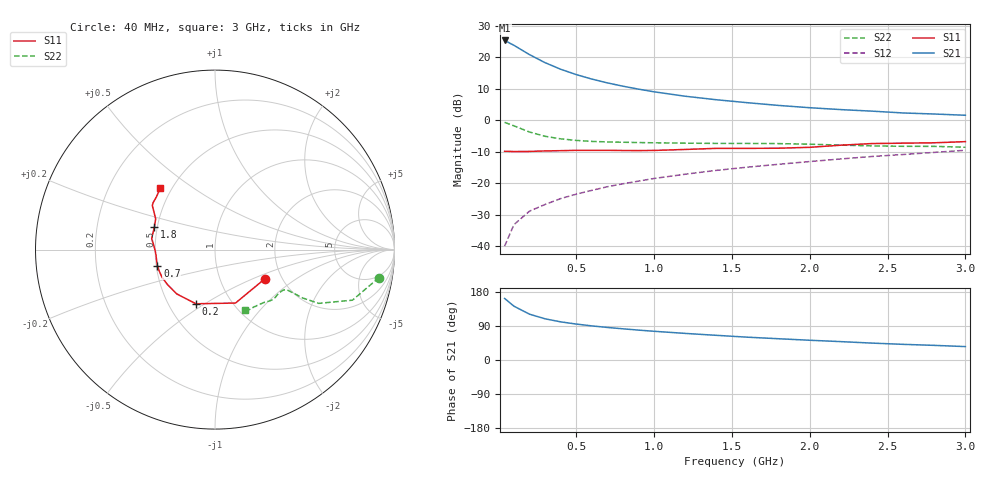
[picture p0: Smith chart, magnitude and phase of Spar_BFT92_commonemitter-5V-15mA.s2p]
! Filename:  BFT92D.S2P  Version:  2.0
! NXP part #: BFT92  Date: May 1990
! Bias condition: Vce=-5V, Ic=-15mA
#  MHz  S  MA  R  50
! Freq  S11  S21  S12  S22  !GUM [dB]
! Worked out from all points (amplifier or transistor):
!   21 points, 40 MHz to 3 GHz, reference 50 ohm
!   highest |S21| = 25.4 dB at 40 MHz (marker M1)
!   |S21| within 3 dB of that: start of sweep to 149.3 MHz
!   unconditionally stable (mu >= 1): 535.4 MHz to 2.211 GHz
!   at 300 MHz: K = 0.84, MSG = 22.5 dB, |S12| = -26.7 dB
!   at 1 GHz: K = 1.09, MAG = 12.0 dB, |S12| = -18.5 dB
!   at 3 GHz: K = 0.91, MSG = 5.6 dB, |S12| = -9.5 dB
!   S11 on the Smith chart (normalised r, x): 40 MHz: 1.64, -0.59; 200 MHz: 0.68, -0.46; 700 MHz: 0.51, -0.10; 1.8 GHz: 0.48, +0.14; 3 GHz: 0.43, +0.37
40  0.322 -30.3  18.55 162.4  0.01 80.9  0.927 -9.7
100  0.319 -69.0  15.53 142.0  0.022 72.1  0.816 -20.2
200  0.32 -109.4  11.05 120.9  0.036 67.1  0.651 -27.4
300  0.326 -130.7  8.228 108.7  0.046 66.8  0.557 -28.9
400  0.329 -144.0  6.473 100.7  0.057 67.9  0.507 -29.0
500  0.333 -152.5  5.323 94.8  0.067 69.1  0.479 -29.1
600  0.333 -159.0  4.52 90.0  0.077 70.0  0.462 -29.2
700  0.333 -164.2  3.929 85.9  0.088 70.7  0.453 -29.6
800  0.331 -169.0  3.482 82.3  0.098 71.4  0.448 -30.0
900  0.33 -173.6  3.125 78.9  0.108 71.6  0.443 -30.6
1000  0.332 -177.7  2.834 75.8  0.119 71.7  0.439 -31.4
1200  0.344 175.2  2.411 70.2  0.139 71.8  0.433 -33.3
1400  0.358 170.1  2.121 65.1  0.16 71.6  0.429 -35.9
1600  0.358 165.4  1.902 60.2  0.18 71.3  0.429 -38.3
1800  0.36 159.8  1.722 56.1  0.2 71.1  0.426 -40.8
2000  0.372 152.7  1.584 52.1  0.221 70.4  0.417 -43.4
2200  0.402 148.0  1.478 48.5  0.243 70.1  0.403 -46.7
2400  0.427 144.9  1.397 44.6  0.266 69.1  0.392 -51.6
2600  0.433 142.7  1.307 41.3  0.286 68.3  0.386 -56.4
2800  0.439 138.0  1.258 38.6  0.309 67.8  0.385 -60.1
3000  0.458 131.9  1.202 35.4  0.334 66.6  0.373 -63.7
